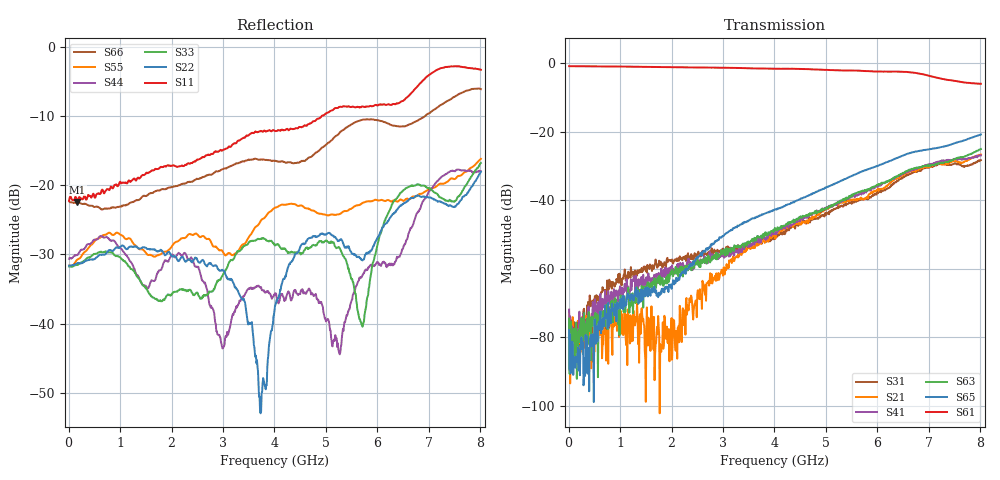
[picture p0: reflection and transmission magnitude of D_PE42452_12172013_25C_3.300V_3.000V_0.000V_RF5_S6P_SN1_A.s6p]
! Device ID: PE42422_06252012
! Dir: z:\David_A\42452\10_28_13_42452_omar_meas\25C\3p300000\RF5
! Serial: 1
! Insertion: A
! Temp: 25C
! VDD: 3.300
! Control_Hi: 3.000
! Control_Lo: 0.000
! Logic State: RF5
! Port 1: RFC
! Port 2: RF1
! Port 3: RF2
! Port 4: RF3
! Port 5: RF4
! Port 6: RF5
! ThroughPath:6-1
! V1 = 3.00
! V2 = 0.00
! V3 = 3.00
! V4 = 0.00
#  Hz  S  RI  R  50
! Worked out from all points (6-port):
!   801 points, 10 MHz to 8.01 GHz, reference 50 ohm
!   strongest paths, dB at 10 MHz, 2.01 GHz, 4.01 GHz, 6.01 GHz, 8.01 GHz:
!     S61: -0.8, -1.1, -1.6, -2.4, -6.0
!     S65: -77.9, -64.6, -42.6, -29.9, -20.8
!     S63: -74.5, -60.2, -48.0, -35.3, -25.0
!     S41: -71.8, -59.0, -49.0, -36.0, -26.9
!     S21: -73.3, -86.5, -51.2, -36.6, -26.6
!     S31: -86.0, -57.3, -51.2, -37.9, -28.3
!   lowest |S11| = -22.4 dB at 170 MHz (marker M1), VSWR 1.16, Z = 57.9 - j2.05 ohm
!   |S11| at or under -10 dB: start of sweep to 4.923 GHz
